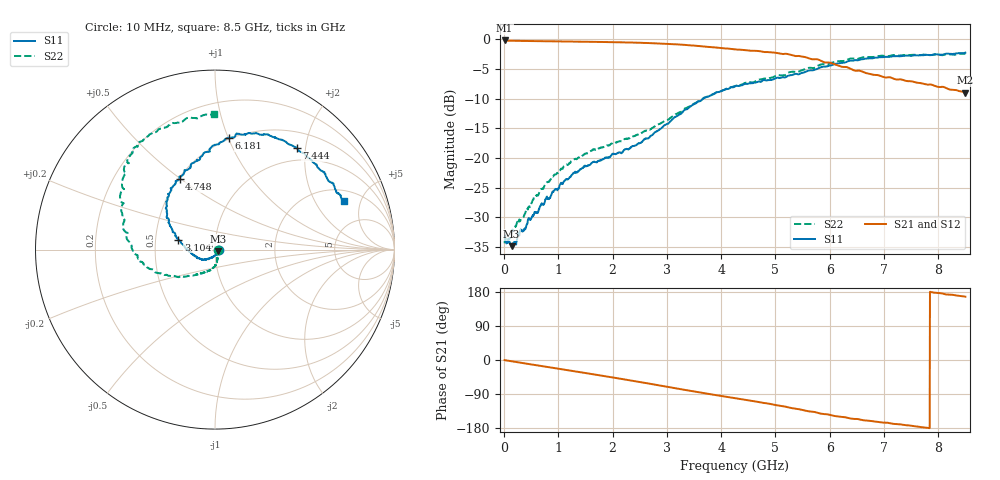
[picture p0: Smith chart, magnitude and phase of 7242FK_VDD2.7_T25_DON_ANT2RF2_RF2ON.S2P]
!Agilent Technologies,E5071C,MY46417908,A.11.23
!Date: Wed Dec 09 15:39:13 2020
!Data & Calibration Information:
!Freq	S11:SOLT2(ON)	S21:SOLT2(ON)	S12:SOLT2(ON)	S22:SOLT2(ON)
!PortZ  Port1:50+j0  Port2:50+j0
!Above PortZ is port z conversion or system Z0 setting when saving the data.
!When reading, reference impedance value at option line is always used.
# Hz S dB R 50
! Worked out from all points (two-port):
!   1601 points, 10 MHz to 8.5 GHz, reference 50 ohm
!   highest |S21| = -0.23 dB at 10 MHz (marker M1); lowest = -9.0 dB at 8.5 GHz (marker M2)
!   |S21| within 3 dB of the highest: start of sweep to 5.616 GHz
!   lowest |S11| = -34.8 dB at 137.3 MHz (marker M3), VSWR 1.04, Z = 51.5 - j1.01 ohm
!   |S11| at or under -10 dB: start of sweep to 3.667 GHz
!   |S22| runs from -34.3 to -2.4 dB; largest |S21 - S12| = 0.0052
!   S11 on the Smith chart (normalised r, x): 10 MHz: 1.04, -0.00; 3.104 GHz: 0.66, +0.08; 4.748 GHz: 0.51, +0.50; 6.181 GHz: 0.49, +1.01; 7.444 GHz: 0.76, +1.83; 8.5 GHz: 2.71, +3.57
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1e7  -33.31 -1.6  -0.23 -0.4  -0.23 -0.4  -34.34 -9.5
1.3735e8  -34.83 -32.6  -0.27 -3.3  -0.28 -3.3  -32.52 -31.5
1.957188e8  -34.11 -42.1  -0.29 -4.7  -0.29 -4.7  -31.65 -41.6
2.912312e8  -32.38 -62.7  -0.29 -6.9  -0.30 -6.9  -30.64 -52.9
5.565438e8  -29.22 -92.3  -0.34 -12.9  -0.34 -12.9  -26.54 -73.0
7.794062e8  -26.74 -108.2  -0.36 -18.0  -0.36 -17.9  -24.17 -79.4
1.108394e9  -23.89 -127.7  -0.40 -25.4  -0.40 -25.4  -21.35 -87.2
1.426769e9  -21.77 -137.2  -0.44 -32.8  -0.44 -32.8  -19.68 -97.4
2.164338e9  -19.15 -159.0  -0.54 -50.0  -0.54 -50.0  -17.20 -115.0
2.843538e9  -15.37 174.7  -0.72 -66.6  -0.72 -66.7  -14.33 -131.2
3.103544e9  -13.48 164.6  -0.84 -73.2  -0.84 -73.2  -13.02 -137.6
3.692538e9  -9.83 146.4  -1.26 -87.7  -1.26 -87.7  -9.87 -154.7
4.255e9  -7.94 129.8  -1.73 -100.8  -1.73 -100.8  -7.90 -167.8
4.748481e9  -7.10 116.6  -2.10 -112.6  -2.08 -112.6  -6.75 -179.8
5.263188e9  -6.12 105.4  -2.60 -125.8  -2.58 -125.8  -5.55 166.4
5.671769e9  -5.27 94.2  -3.38 -136.3  -3.34 -136.3  -4.85 153.2
6.181169e9  -4.04 82.8  -4.51 -149.5  -4.52 -149.2  -3.70 140.7
6.690569e9  -3.27 70.8  -5.75 -160.0  -5.77 -159.8  -3.03 132.0
7.088538e9  -2.99 61.4  -6.41 -166.2  -6.46 -166.4  -2.85 126.8
7.444056e9  -2.78 51.3  -7.08 -172.3  -7.08 -172.3  -2.69 120.9
7.9057e9  -2.60 36.2  -7.75 178.1  -7.76 178.2  -2.63 110.6
8.5e9  -2.29 20.5  -9.02 167.1  -9.12 167.1  -2.43 90.5
